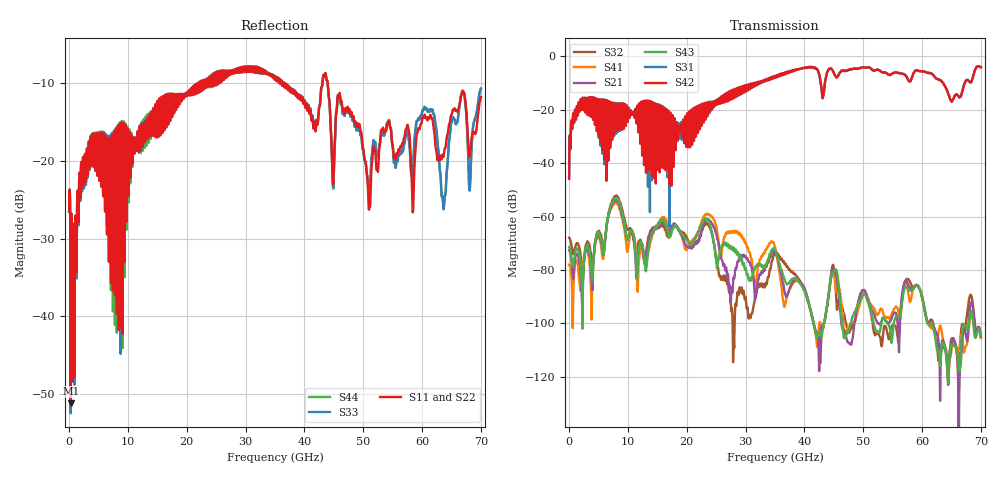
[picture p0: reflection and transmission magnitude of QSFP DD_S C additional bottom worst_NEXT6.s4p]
! AWR Design Environment (8415) Thu Dec 20 16:37:10 2018
! Document = 'CHANNEL TEST'
! nPorts: 4, nXvals: 7001
# HZ S DB R 50
!Freq DBS11 AngS11 DBS12 AngS12 DBS13 AngS13 DBS14 AngS14
!	DBS21 AngS21 DBS22 AngS22 DBS23 AngS23 DBS24 AngS24
!	DBS31 AngS31 DBS32 AngS32 DBS33 AngS33 DBS34 AngS34
!	DBS41 AngS41 DBS42 AngS42 DBS43 AngS43 DBS44 AngS44
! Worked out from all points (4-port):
!   7000 points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, 10 MHz to 70 GHz, reference 50 ohm
!   strongest paths, dB at 10 MHz, 17.51 GHz, 35.01 GHz, 52.51 GHz, 70 GHz:
!     S42: -45.8, -24.5, -7.4, -5.0, -4.0
!     S31: -45.8, -25.1, -7.4, -5.0, -4.0
!     S43: -71.4, -64.9, -72.5, -103.1, -104.9
!     S21: -72.6, -63.3, -73.1, -99.8, -105.1
!     S41: -78.0, -64.3, -71.3, -96.6, -105.4
!     S32: -67.9, -63.5, -73.8, -103.7, -104.6
!   lowest |S11| = -51.2 dB at 280 MHz (marker M1), VSWR 1.01, Z = 50.1 + j0.257 ohm
!   |S11| at or under -10 dB: start of sweep to 21.8 GHz; 36.76 GHz to 43.07 GHz (6.307 GHz wide, 15.8 % of centre); 43.96 GHz to end of sweep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
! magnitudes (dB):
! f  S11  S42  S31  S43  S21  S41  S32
! 10 MHz  -26.4  -45.8  -45.8  -71.4  -72.6  -78.0  -67.9
! 280 MHz  -51.2  -30.0  -30.2  -73.2  -74.4  -79.8  -69.4
! 7.93 GHz  -16.1  -22.9  -22.5  -53.3  -54.0  -55.0  -52.4
! 13.04 GHz  -14.9  -26.2  -26.4  -80.5  -75.9  -75.7  -74.8
! 23.51 GHz  -9.4  -21.7  -21.6  -61.0  -60.9  -58.9  -62.5
! 27.09 GHz  -8.6  -15.7  -15.7  -71.1  -83.4  -65.9  -85.5
! 70 GHz  -11.7  -4.0  -4.0  -104.9  -105.1  -105.4  -104.6
